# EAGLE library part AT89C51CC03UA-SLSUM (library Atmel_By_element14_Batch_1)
Enhanced 8-bit MCU with CAN Controller
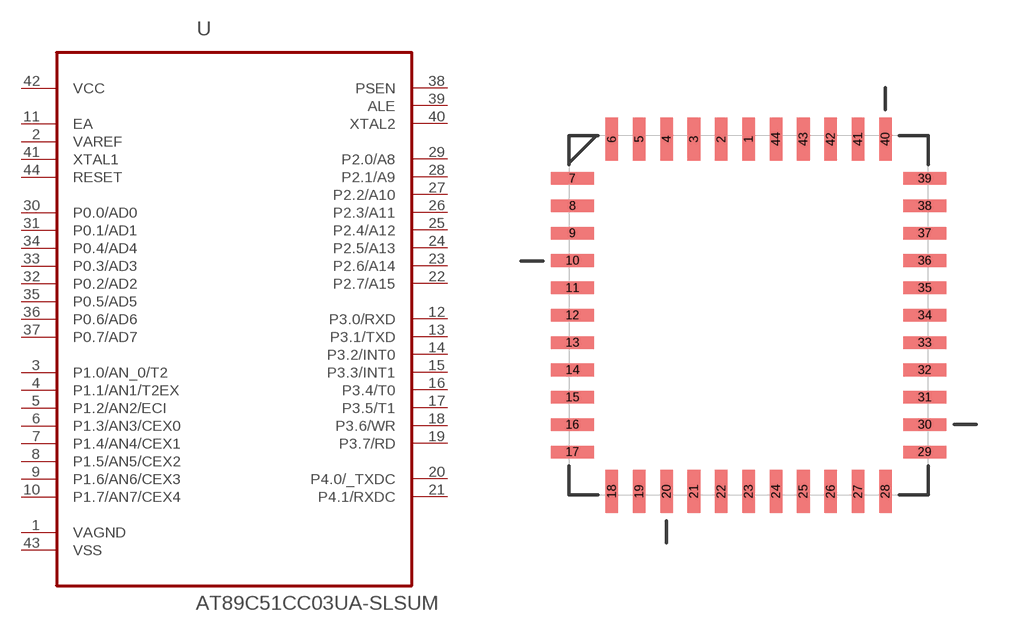
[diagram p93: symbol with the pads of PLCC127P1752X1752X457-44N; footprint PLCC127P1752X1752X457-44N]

Designator prefix U

## AT89C51CC03UA-SLSUM (DESCRIPTION: Enhanced 8-bit MCU with CAN Controller; MPN: AT89C51CC03UA-SLSUM; OC_FARNELL: 1095723; OC_NEWARK: 96K6566; PACKAGE: PLCC-44; SUPPLIER: ATMEL)  [PLCC127P1752X1752X457-44N]
1  VAGND  pas
2  VAREF  in
3  P1.0/AN_0/T2
4  P1.1/AN1/T2EX
5  P1.2/AN2/ECI
6  P1.3/AN3/CEX0
7  P1.4/AN4/CEX1
8  P1.5/AN5/CEX2
9  P1.6/AN6/CEX3
10  P1.7/AN7/CEX4
11  EA  in
12  P3.0/RXD
13  P3.1/TXD
14  P3.2/INT0
15  P3.3/INT1
16  P3.4/T0
17  P3.5/T1
18  P3.6/WR
19  P3.7/RD
20  P4.0/_TXDC
21  P4.1/RXDC
22  P2.7/A15
23  P2.6/A14
24  P2.5/A13
25  P2.4/A12
26  P2.3/A11
27  P2.2/A10
28  P2.1/A9
29  P2.0/A8
30  P0.0/AD0
31  P0.1/AD1
32  P0.2/AD2
33  P0.3/AD3
34  P0.4/AD4
35  P0.5/AD5
36  P0.6/AD6
37  P0.7/AD7
38  PSEN  out
39  ALE  out
40  XTAL2  out
41  XTAL1  in
42  VCC  pwr
43  VSS  pwr
44  RESET  in

## Footprint PLCC127P1752X1752X457-44N (pad centres in mm)
smd 0.584 x 2.007: 1 0,8.179; 2 -1.27,8.179; 3 -2.54,8.179; 4 -3.81,8.179; 5 -5.08,8.179; 6 -6.35,8.179; 18 -6.35,-8.179; 19 -5.08,-8.179; 20 -3.81,-8.179; 21 -2.54,-8.179; 22 -1.27,-8.179; 23 0,-8.179; 24 1.27,-8.179; 25 2.54,-8.179; 26 3.81,-8.179; 27 5.08,-8.179; 28 6.35,-8.179; 40 6.35,8.179; 41 5.08,8.179; 42 3.81,8.179; 43 2.54,8.179; 44 1.27,8.179
smd 2.007 x 0.584: 7 -8.179,6.35; 8 -8.179,5.08; 9 -8.179,3.81; 10 -8.179,2.54; 11 -8.179,1.27; 12 -8.179,0; 13 -8.179,-1.27; 14 -8.179,-2.54; 15 -8.179,-3.81; 16 -8.179,-5.08; 17 -8.179,-6.35; 29 8.179,-6.35; 30 8.179,-5.08; 31 8.179,-3.81; 32 8.179,-2.54; 33 8.179,-1.27; 34 8.179,0; 35 8.179,1.27; 36 8.179,2.54; 37 8.179,3.81; 38 8.179,5.08; 39 8.179,6.35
